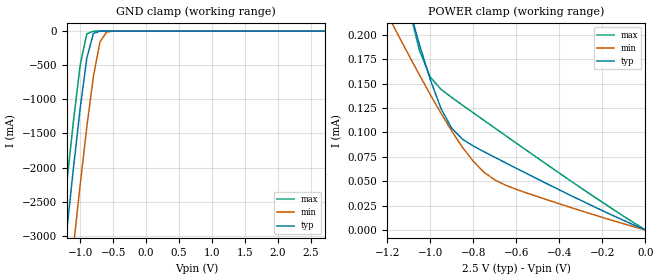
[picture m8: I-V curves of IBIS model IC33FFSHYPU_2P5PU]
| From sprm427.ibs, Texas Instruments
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|   Model IC33FFSHYPU_2P5PU
[Model]   IC33FFSHYPU_2P5PU
Model_type   Input
Polarity   Non-Inverting
Vinl =   0.7500V
Vinh =   1.7500V
C_comp   2.1510pF   2.1423pF   2.1675pF
[Temperature Range]   25.0000   0.1250k   -40.0000
[Voltage Range]   2.5000V   2.3000V   2.7000V
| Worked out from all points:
|   GND clamp passes 1 mA (typ) near -0.69 V on its own axis
|   POWER clamp passes 1 mA (typ) near -1.95 V on its own axis
[GND_clamp]
| voltage   I(typ)   I(min)   I(max)
-2.5V     -15.45A    -16.55A    -14.8A
-1.3V     -3.808A    -4.968A    -3.114A
-1.2V     -2.88A     -4.039A    -2.185A
-1.1V     -1.977A    -3.127A    -1.292A
-1V       -1.123A    -2.241A    -489.8mA
-900mV    -393.5mA   -1.402A    -39.38mA
-800mV    -34.13mA   -660.7mA   -2.513mA
-700mV    -1.135mA   -156.4mA   -340.7uA
-600mV    -112.1uA   -13.16mA   -121.7uA
-400mV    -69.03uA   -89.1uA    -108.1uA
2.72V     0A         0A         0A
[POWER_clamp]
| voltage   I(typ)   I(min)   I(max)
-2.5V     1.524mA    807.6uA    2.104mA
-1.2V     313.7uA    221.8uA    342.9uA
-1.15V    271uA      200.5uA    283.6uA
-1.1V     229.6uA    179.6uA    229.1uA
-1.05V    190.3uA    159.1uA    184.3uA
-1V       154.5uA    139.1uA    156.9uA
-950mV    124.7uA    119.8uA    144.3uA
-900mV    104.3uA    101.6uA    135.9uA
-850mV    93.13uA    84.86uA    128uA
-750mV    80.25uA    59.22uA    112.4uA
-650mV    68.9uA     45.97uA    96.83uA
0V        157.4pA    1.102nA    165.8pA
